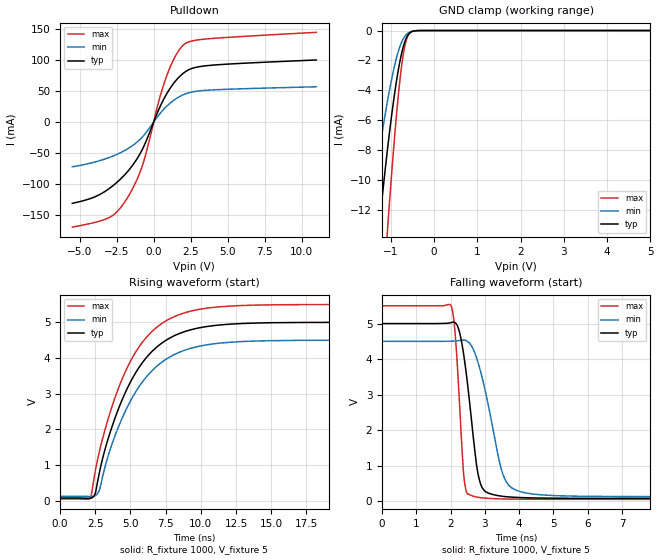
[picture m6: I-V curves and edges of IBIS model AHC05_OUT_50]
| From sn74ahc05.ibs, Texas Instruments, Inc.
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[Model]   AHC05_OUT_50
Model_type  Open_drain
Enable   Active-Low
Vref =   5
Rref =   1000
Cref =   50p
Vmeas =   2.5
| variable   typ   min   max
C_comp   2.08pF   1.52pF   2.41pF
| C_pulldown   3.81pF   2.17pF   6.07pF
| C_tri-state   2.08pF   1.52pF   2.41pF
[Temperature Range]   40   100   -40
| Ambient temperature   25   85   -40
[Voltage range]   5   4.5   5.5
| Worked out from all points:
|   slope of the pulldown table from 0 to 0.75 V, typ, clamps not added: 18.8 ohm
|   GND clamp passes 1 mA (typ) near -0.70 V on its own axis
|   rising waveform, R_fixture 1000, V_fixture 5: 20-80 % time 3.2ns typ, 3.26ns min, 3.14ns max; typ from 0.079 V to 5 V
|   falling waveform, R_fixture 1000, V_fixture 5: 20-80 % time 352ps typ, 571ps min, 196ps max; typ from 5 V to 0.079 V
[GND Clamp]
| AHC05_OUT_50
|   Voltage   I(typ)   I(min)   I(max)
-5.5V     -200.4mA   -131.5mA   -251.9mA
-1.545V   -21.83mA   -13.78mA   -34.66mA
-1.49V    -20.02mA   -12.6mA    -32.01mA
-1.265V   -13.08mA   -8.076mA   -21.55mA
-1.085V   -8.206mA   -4.892mA   -13.79mA
-1.06V    -7.585mA   -4.489mA   -12.77mA
-915mV    -4.315mA   -2.403mA   -7.271mA
-840mV    -2.903mA   -1.55mA    -4.812mA
-765mV    -1.745mA   -897.7uA   -2.76mA
-655mV    -608.9uA   -322.7uA   -807.4uA
-545mV    -126.2uA   -86.8uA    -124.8uA
5V        57.09nA    3.594nA    534.3nA
[Pulldown]
| AHC05_OUT_50
|   Voltage   I(typ)   I(min)   I(max)
-5.5V     -131.1mA   -72.19mA   -169.5mA
-4.045V   -121.3mA   -64.89mA   -162.2mA
-2.97V    -106.6mA   -56.88mA   -153.5mA
-2.39V    -95.25mA   -51.14mA   -142.4mA
-1.755V   -79.61mA   -43.12mA   -121.3mA
-735mV    -42.64mA   -23.43mA   -68.24mA
350mV     20.45mA    11.37mA    33.9mA
890mV     45.88mA    25.64mA    74.98mA
1.485V    66.36mA    37.18mA    106.9mA
2.05V     79.45mA    44.45mA    125mA
3.725V    91.14mA    51.39mA    134.3mA
11V       100mA      56.83mA    144.6mA
[Ramp]
| AHC05_OUT_50
| variable   typ   min   max
dV/dt_r   2.96/3.20E-09   2.63/3.26E-09   3.27/3.14E-09
dV/dt_f   2.97/3.58E-10   2.64/5.78E-10   3.29/2.00E-10
R_load = 1000
[Rising Waveform]
| AHC05_OUT_50
R_fixture =   1000
C_fixture =   0
L_fixture =   0
V_fixture =   5
V_fixture_min = 4.5
V_fixture_max = 5.5
|   Time   V(typ)   V(min)   V(max)
0s        79.2mV     128.4mV    52.12mV
2.135ns   72.62mV    122.3mV    74.29mV
2.485ns   199.7mV    147.2mV    804.4mV
2.755ns   723.7mV    266.3mV    1.322V
3.33ns    1.634V     1.151V     2.187V
4.97ns    3.307V     2.774V     3.888V
6.735ns   4.261V     3.722V     4.817V
9.035ns   4.763V     4.242V     5.287V
15.13ns   4.989V     4.487V     5.49V
50ns      5V         4.5V       5.499V
[Falling Waveform]
| AHC05_OUT_50
R_fixture =   1000
C_fixture =   0
L_fixture =   0
V_fixture =   5
V_fixture_min = 4.5
V_fixture_max = 5.5
|   Time   V(typ)   V(min)   V(max)
0s        5V         4.5V       5.499V
2.02ns    5.028V     4.503V     5.488V
2.145ns   5.014V     4.51V      4.563V
2.365ns   4.232V     4.533V     948.2mV
2.415ns   3.899V     4.531V     474.7mV
2.755ns   1.029V     4.04V      117.6mV
2.905ns   409.5mV    3.537V     95.44mV
3.6ns     128.4mV    588.3mV    62.1mV
4.67ns    87.47mV    175.8mV    53.81mV
50ns      79.2mV     128.4mV    52.12mV
